PROGRAM ModbusMaster
VAR
	iSlaveID:USINT:=1;
	bPcCOM:BOOL;

	MB_EL6x22B	:ModbusRtuMaster_KL6x22B;
	MB_PcCOM	:ModbusRtuMaster_PcCOM;

	MBData_Read : ARRAY[0..9] OF WORD;	(* Read from Modbus  Slaves *)
	MBdata_Write : ARRAY[0..9] OF WORD;	(* Write to  Modbus  Slaves *)
	bRead: BOOL;
	bWrite: BOOL;
	iReadMBAddr:WORD:=1;
	iWriteMBAddr:WORD:=1;
	iReadQty:WORD:=1;
	iWriteQty:WORD:=1;

	fbTrigerWrite:R_TRIG;
	nErrID:MODBUS_ERRORS;
END_VAR

MB_EL6x22B.ReadRegs(
	UnitID:=iSlaveID,
	Quantity:=iReadQty ,
	MBAddr:=iReadMBAddr ,
	cbLength:= iReadQty*2,
	pMemoryAddr:= ADR(MBData_Read),
	Execute:=bRead ,
	Timeout:=t#500ms ,
	BUSY=> ,
	Error=> ,
	ErrorId=>nErrID ,
	cbRead=> );


fbTrigerWrite(CLK:=bWrite, Q=> );

MB_EL6x22B.WriteRegs(
	UnitID:= iSlaveID,
	Quantity:=iWriteQty ,
	MBAddr:=iWriteMBAddr ,
	cbLength:= iWriteQty*2,
	pMemoryAddr:= ADR(MBData_Write),
	Execute:=fbTrigerWrite.Q,
	Timeout:=t#500ms ,
	BUSY=> ,
	Error=> ,
	ErrorId=>nErrID ,
	cbRead=> );

END_PROGRAM
